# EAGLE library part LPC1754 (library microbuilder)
LPC1754 100 MHz 32-bit ARM Cortex-M3 microcontroller - 128 kB Flash, 32 kB SRAM, USB Device/Host/OTG, CAN, DAC, RTC Digikey: 568-4790-ND
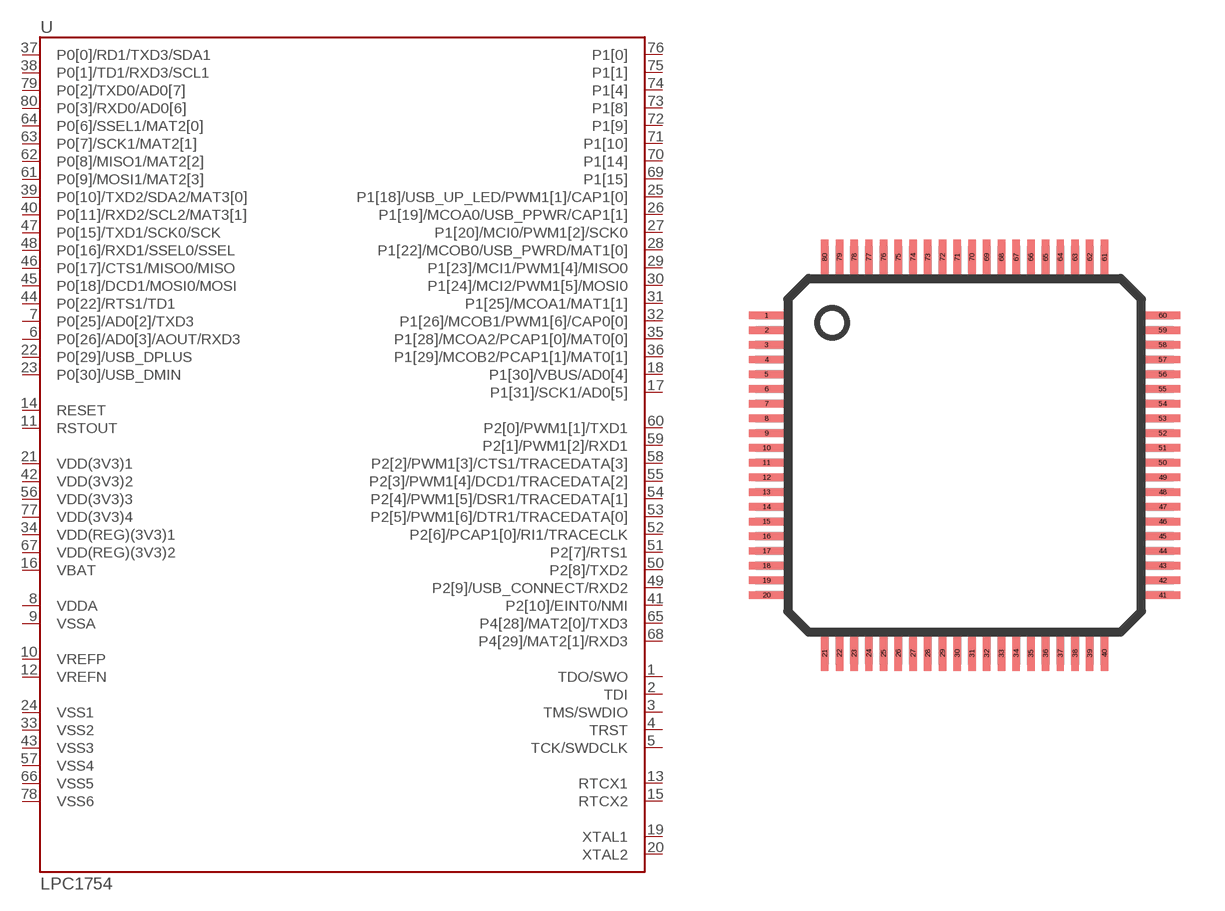
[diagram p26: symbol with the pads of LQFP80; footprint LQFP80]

Designator prefix U

## LPC1754  [LQFP80]
1  TDO/SWO  out
2  TDI  in
3  TMS/SWDIO
4  TRST
5  TCK/SWDCLK
6  P0[26]/AD0[3]/AOUT/RXD3
7  P0[25]/AD0[2]/TXD3
8  VDDA  pwr
9  VSSA  pwr
10  VREFP  in
11  RSTOUT  out
12  VREFN  in
13  RTCX1  in
14  RESET  in
15  RTCX2  out
16  VBAT  pwr
17  P1[31]/SCK1/AD0[5]
18  P1[30]/VBUS/AD0[4]
19  XTAL1  in
20  XTAL2  out
21  VDD(3V3)1  pwr
22  P0[29]/USB_DPLUS
23  P0[30]/USB_DMIN
24  VSS1  pwr
25  P1[18]/USB_UP_LED/PWM1[1]/CAP1[0]
26  P1[19]/MCOA0/USB_PPWR/CAP1[1]
27  P1[20]/MCI0/PWM1[2]/SCK0
28  P1[22]/MCOB0/USB_PWRD/MAT1[0]
29  P1[23]/MCI1/PWM1[4]/MISO0
30  P1[24]/MCI2/PWM1[5]/MOSI0
31  P1[25]/MCOA1/MAT1[1]
32  P1[26]/MCOB1/PWM1[6]/CAP0[0]
33  VSS2  pwr
34  VDD(REG)(3V3)1  pwr
35  P1[28]/MCOA2/PCAP1[0]/MAT0[0]
36  P1[29]/MCOB2/PCAP1[1]/MAT0[1]
37  P0[0]/RD1/TXD3/SDA1
38  P0[1]/TD1/RXD3/SCL1
39  P0[10]/TXD2/SDA2/MAT3[0]
40  P0[11]/RXD2/SCL2/MAT3[1]
41  P2[10]/EINT0/NMI
42  VDD(3V3)2  pwr
43  VSS3  pwr
44  P0[22]/RTS1/TD1
45  P0[18]/DCD1/MOSI0/MOSI
46  P0[17]/CTS1/MISO0/MISO
47  P0[15]/TXD1/SCK0/SCK
48  P0[16]/RXD1/SSEL0/SSEL
49  P2[9]/USB_CONNECT/RXD2
50  P2[8]/TXD2
51  P2[7]/RTS1
52  P2[6]/PCAP1[0]/RI1/TRACECLK
53  P2[5]/PWM1[6]/DTR1/TRACEDATA[0]
54  P2[4]/PWM1[5]/DSR1/TRACEDATA[1]
55  P2[3]/PWM1[4]/DCD1/TRACEDATA[2]
56  VDD(3V3)3  pwr
57  VSS4  pwr
58  P2[2]/PWM1[3]/CTS1/TRACEDATA[3]
59  P2[1]/PWM1[2]/RXD1
60  P2[0]/PWM1[1]/TXD1
61  P0[9]/MOSI1/MAT2[3]
62  P0[8]/MISO1/MAT2[2]
63  P0[7]/SCK1/MAT2[1]
64  P0[6]/SSEL1/MAT2[0]
65  P4[28]/MAT2[0]/TXD3
66  VSS5  pwr
67  VDD(REG)(3V3)2  pwr
68  P4[29]/MAT2[1]/RXD3
69  P1[15]
70  P1[14]
71  P1[10]
72  P1[9]
73  P1[8]
74  P1[4]
75  P1[1]
76  P1[0]
77  VDD(3V3)4  pwr
78  VSS6  pwr
79  P0[2]/TXD0/AD0[7]
80  P0[3]/RXD0/AD0[6]

## Footprint LQFP80 (pad centres in mm)
LQFP80 Low profile Quad Flat Package 12x12x1.4 mm
smd 1.2 x 0.254: 1 -6.725,4.75; 2 -6.725,4.25; 3 -6.725,3.75; 4 -6.725,3.25; 5 -6.725,2.75; 6 -6.725,2.25; 7 -6.725,1.75; 8 -6.725,1.25; 9 -6.725,0.75; 10 -6.725,0.25; 11 -6.725,-0.25; 12 -6.725,-0.75; 13 -6.725,-1.25; 14 -6.725,-1.75; 15 -6.725,-2.25; 16 -6.725,-2.75; 17 -6.725,-3.25; 18 -6.725,-3.75; 19 -6.725,-4.25; 20 -6.725,-4.75; 41 6.725,-4.75; 42 6.725,-4.25; 43 6.725,-3.75; 44 6.725,-3.25; 45 6.725,-2.75; 46 6.725,-2.25; 47 6.725,-1.75; 48 6.725,-1.25; 49 6.725,-0.75; 50 6.725,-0.25; 51 6.725,0.25; 52 6.725,0.75; 53 6.725,1.25; 54 6.725,1.75; 55 6.725,2.25; 56 6.725,2.75; 57 6.725,3.25; 58 6.725,3.75; 59 6.725,4.25; 60 6.725,4.75
smd 0.254 x 1.2: 21 -4.75,-6.725; 22 -4.25,-6.725; 23 -3.75,-6.725; 24 -3.25,-6.725; 25 -2.75,-6.725; 26 -2.25,-6.725; 27 -1.75,-6.725; 28 -1.25,-6.725; 29 -0.75,-6.725; 30 -0.25,-6.725; 31 0.25,-6.725; 32 0.75,-6.725; 33 1.25,-6.725; 34 1.75,-6.725; 35 2.25,-6.725; 36 2.75,-6.725; 37 3.25,-6.725; 38 3.75,-6.725; 39 4.25,-6.725; 40 4.75,-6.725; 61 4.75,6.725; 62 4.25,6.725; 63 3.75,6.725; 64 3.25,6.725; 65 2.75,6.725; 66 2.25,6.725; 67 1.75,6.725; 68 1.25,6.725; 69 0.75,6.725; 70 0.25,6.725; 71 -0.25,6.725; 72 -0.75,6.725; 73 -1.25,6.725; 74 -1.75,6.725; 75 -2.25,6.725; 76 -2.75,6.725; 77 -3.25,6.725; 78 -3.75,6.725; 79 -4.25,6.725; 80 -4.75,6.725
